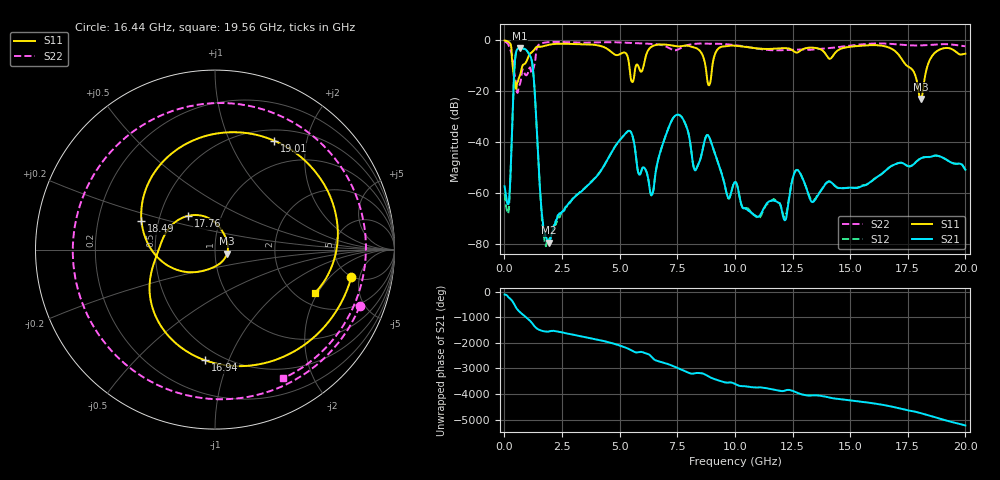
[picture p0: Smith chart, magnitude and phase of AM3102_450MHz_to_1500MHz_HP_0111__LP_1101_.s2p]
!Agilent Technologies,E8364B,MY43040894,A.07.50.67
!Agilent E8364B: A.07.50.67
!Date: Thursday, January 11, 2018 05:54:33
!Correction: S11(Full 2 Port(1,2))
!S21(Full 2 Port(1,2))
!S12(Full 2 Port(1,2))
!S22(Full 2 Port(1,2))
!S2P File: Measurements: S11, S21, S12, S22:
# Hz S  dB  R 50
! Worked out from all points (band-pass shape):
!   1601 points, 10 MHz to 20 GHz, reference 50 ohm
!   highest |S21| = -3.02 dB at 672.2 MHz (marker M1); lowest = -79.5 dB at 1.934 GHz (marker M2)
!   |S21| within 3 dB of the highest: 482.2 MHz to 1.111 GHz (628.6 MHz wide, 78.9 % of centre)
!   lowest |S11| = -23.0 dB at 18.06 GHz (marker M3), VSWR 1.15, Z = 57.2 - j2.55 ohm
!   |S11| at or under -10 dB: 360.3 MHz to 783.3 MHz (423 MHz wide, 74 % of centre); 8.723 GHz to 9.023 GHz (299.9 MHz wide, 3.38 % of centre); 17.47 GHz to 18.36 GHz (891.1 MHz wide, 4.97 % of centre)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
!   |S22| runs from -20.6 to -0.5 dB; largest |S21 - S12| = 0.002
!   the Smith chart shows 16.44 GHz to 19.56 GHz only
!   S11 on the Smith chart (normalised r, x): 16.44 GHz: 4.91, -3.78; 16.94 GHz: 0.41, -0.83; 17.76 GHz: 0.70, +0.28; 18.49 GHz: 0.40, +0.16; 19.01 GHz: 0.64, +1.48; 19.56 GHz: 2.50, -1.90
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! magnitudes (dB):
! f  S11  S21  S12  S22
! 10 MHz  -0.1  -57.3  -60.4  -0.5
! 184.9 MHz  -0.6  -64.1  -67.1  -1.9
! 459.8 MHz  -16.9  -8.0  -8.0  -14.1
! 672.2 MHz  -13.9  -3.0  -3.0  -17.2
! 1.197 GHz  -4.7  -8.4  -8.4  -12.7
! 1.659 GHz  -2.4  -70.6  -73.5  -1.1
! 1.934 GHz  -1.8  -79.5  -78.2  -0.7
! 3.346 GHz  -1.5  -59.3  -59.0  -0.9
! 5.357 GHz  -6.7  -35.7  -35.7  -1.0
! 6.682 GHz  -1.7  -46.5  -46.5  -1.6
! 7.569 GHz  -2.4  -29.3  -29.3  -3.4
! 10.01 GHz  -2.1  -55.7  -55.6  -1.9
! 13.34 GHz  -2.9  -63.5  -63.0  -3.7
! 16.44 GHz  -2.2  -52.0  -51.9  -1.3
! 16.68 GHz  -2.8  -50.0  -50.1  -1.3
! 16.94 GHz  -4.2  -48.7  -48.7  -1.5
! 17.76 GHz  -12.4  -48.6  -48.5  -2.0
! 18.06 GHz  -23.0  -46.4  -46.3  -2.0
! 18.49 GHz  -7.1  -45.8  -45.8  -1.8
! 19.01 GHz  -3.2  -46.1  -46.1  -1.5
! 19.56 GHz  -4.3  -48.5  -48.5  -1.8
! 20 GHz  -5.2  -50.8  -50.8  -2.3
